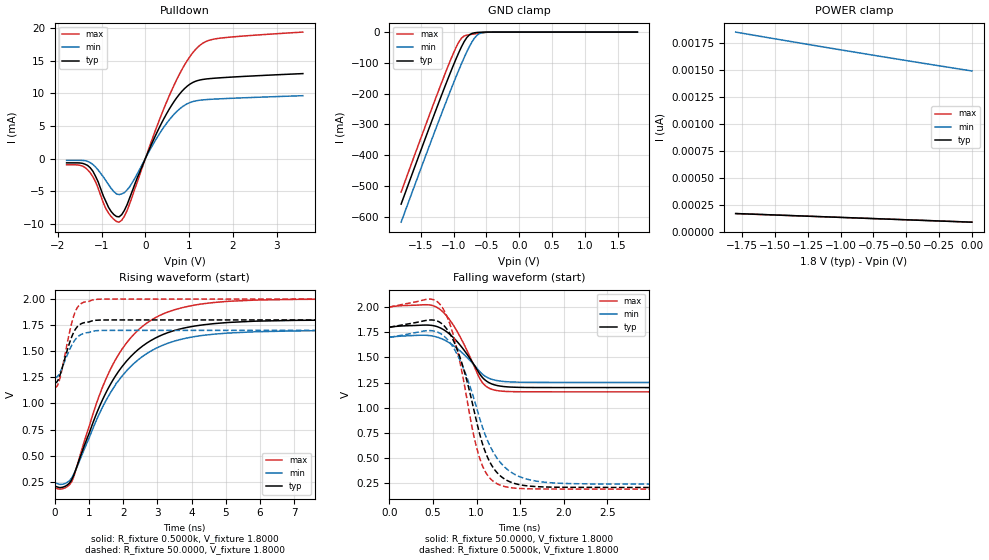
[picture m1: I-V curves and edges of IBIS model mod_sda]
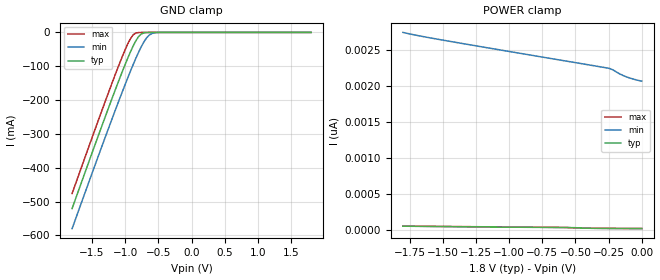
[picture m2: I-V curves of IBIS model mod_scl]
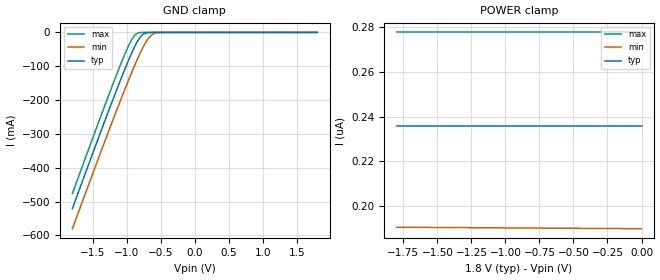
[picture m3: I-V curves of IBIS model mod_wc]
| IBIS (I/O, Buffer, Information, Specification) Model, officially
| electronic behavioral standard for Buffer structures of digital pins.
[IBIS ver]  4.0
[File name] m24c16_g1_tssop8.ibs
[File Rev]  0
[Date]   18 March 2015
[Source]   CAD & Design Services (Catania) - STMicroelectronics
[Notes]
   (Note1)  This IBIS model includes the TSSOP8 package data
   (Note2)  This IBIS model has some Notes about the non-monotonicity
   of the I-V curves, but they are not indicative of problems
   inside the model;
[Copyright] (c) 2015 STMicroelectronics
|   Component M24C16
[Component] M24C16
[Manufacturer] STMicroelectronics
[Package]
| variable  typ   min   max
R_pkg   0.0   0.0   0.0
L_pkg   0.0H   0.0H   0.0H
C_pkg   0.0F   0.0F   0.0F
[Pin]  signal_name   model_name   R_pin   L_pin   C_pin
1   NC   NC   NA   NA   NA
2   NC   NC   NA   NA   NA
3   NC   NC   NA   NA   NA
4   VSS   GND   NA   NA   NA
5   SDA   mod_sda   NA   NA   NA
6   SCL   mod_scl   NA   NA   NA
7   WCN   mod_wc   NA   NA   NA
8   VCC   POWER   NA   NA   NA
[Package Model]  182696_TSSOP8
[Define Package Model]  182696_TSSOP8
[Manufacturer]  STMicroelectronics
[OEM]  STMicroelectronics
[Description]  8 pin TSSOP package
[Number Of Pins]  8
[Pin Numbers]
|Pin Num   Terminal Name
1   | net1
2   | net2
3   | net3
4   | net4_GND
5   | net5
6   | net6
7   | net7
8   | net8_VDD
[Model Data]
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[End Model Data]
[End Package Model]
| Models and submodels in the file (3): mod_sda (I/O_open_drain), mod_scl (Input), mod_wc (Input)
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|   Model mod_sda
[Model]   mod_sda
Model_type I/O_open_drain
Polarity   Non-Inverting
Vinl   =   0.540V
Vinh   =   1.260V
Vmeas  =   0.900V
Cref   =   10pF
Rref   =   1k
Vref   =   1.800V
C_comp   2.668pF   2.547pF   2.925pF
[Temperature Range]  25.0000   0.1050k   -40.0000
[Voltage Range]   1.8000V   1.7000V   2.0000V
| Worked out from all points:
|   slope of the pulldown table from 0 to 0.27 V, typ, clamps not added: 66.3 ohm
|   GND clamp passes 1 mA (typ) near -0.63 V on its own axis
|   rising waveform, R_fixture 0.5000k, V_fixture 1.8000: 20-80 % time 1.53ns typ, 1.58ns min, 1.46ns max; typ from 0.207 V to 1.8 V
|   rising waveform, R_fixture 50.0000, V_fixture 1.8000: 20-80 % time 352ps typ, 384ps min, 337ps max; typ from 1.2 V to 1.8 V
|   falling waveform, R_fixture 50.0000, V_fixture 1.8000: 20-80 % time 297ps typ, 311ps min, 292ps max; typ from 1.8 V to 1.2 V
|   falling waveform, R_fixture 0.5000k, V_fixture 1.8000: 20-80 % time 300ps typ, 367ps min, 258ps max; typ from 1.8 V to 0.207 V
[Pulldown]
|Voltage   I(typ)   I(min)   I(max)
-1.8V     -665.8uA   -275.1uA   -956.4uA
-1.44V    -730.5uA   -283.4uA   -1.147mA
-1.26V    -1.416mA   -626uA     -2.177mA
-900mV    -6.632mA   -3.421mA   -7.74mA
-600mV    -8.957mA   -5.543mA   -9.785mA
-420mV    -7.139mA   -4.839mA   -8.038mA
60mV      953.5uA    767.3uA    1.16mA
480mV     6.822mA    5.362mA    8.599mA
840mV     10.37mA    7.928mA    13.73mA
1.14V     11.86mA    8.85mA     16.72mA
1.62V     12.37mA    9.153mA    18.42mA
3.6V      13.06mA    9.66mA     19.44mA
[GND_clamp]
|Voltage   I(typ)   I(min)   I(max)
-1.8V     -559.4mA   -618.2mA   -520.2mA
-1.2V     -214.3mA   -274.2mA   -173.7mA
-1.04V    -126.9mA   -186.2mA   -87.22mA
-960mV    -85.5mA    -143.6mA   -48.31mA
-880mV    -47.65mA   -102.7mA   -19.45mA
-800mV    -17.95mA   -64.52mA   -9.981mA
-760mV    -8.981mA   -47.2mA    -8.395mA
-720mV    -4.357mA   -31.76mA   -7.048mA
-640mV    -1.164mA   -9.757mA   -4.512mA
-560mV    -259.3uA   -1.789mA   -2.186mA
-440mV    -32.94uA   -178.5uA   -105.7uA
1.8V      87.14pA    1.509nA    78.96pA
[POWER_clamp]
|Voltage   I(typ)   I(min)   I(max)
-1.8V     167.6pA    1.851nA    166.7pA
-960mV    129.9pA    1.678nA    129.9pA
-480mV    108.5pA    1.583nA    108.8pA
0V        87.14pA    1.49nA     87.73pA
[Ramp]
| variable   typ   min   max
dV/dt_r   0.3599/0.4505n   0.2623/0.5115n   0.5053/0.3901n
dV/dt_f   0.3599/0.3419n   0.2623/0.3879n   0.5053/0.3191n
R_load = 50.0000
[Rising Waveform]   | New Temp 105 (min)
R_fixture= 0.5000k
V_fixture= 1.8000
V_fixture_min= 1.7000
V_fixture_max= 2.0000
|time   V(typ)   V(min)   V(max)
0s        207.5mV    240.5mV    191.1mV
310ps     206.8mV    234mV      192.3mV
510ps     279.3mV    293.7mV    260.1mV
1.27ns    941.6mV    877.8mV    1.047V
1.8ns     1.275V     1.193V     1.433V
2.33ns    1.485V     1.387V     1.668V
2.93ns    1.624V     1.523V     1.82V
3.77ns    1.721V     1.62V      1.921V
5.08ns    1.776V     1.674V     1.979V
10ns      1.8V       1.699V     2V
[Rising Waveform]
R_fixture= 50.0000
V_fixture= 1.8000   | New Temp (105)
V_fixture_min= 1.7000
V_fixture_max= 2.0000
|time   V(typ)   V(min)   V(max)
0s        1.2V       1.251V     1.158V
70ps      1.21V      1.255V     1.168V
150ps     1.269V     1.296V     1.24V
230ps     1.355V     1.355V     1.355V
450ps     1.597V     1.527V     1.709V
530ps     1.665V     1.577V     1.811V
610ps     1.714V     1.616V     1.887V
770ps     1.763V     1.66V      1.957V
1.11ns    1.792V     1.692V     1.992V
10ns      1.8V       1.7V       2V
[Falling Waveform]
R_fixture= 50.0000   | New Temp 105 (min)
V_fixture= 1.8000
V_fixture_min= 1.7000
V_fixture_max= 2.0000
|time   V(typ)   V(min)   V(max)
0s        1.8V       1.7V       2V
440ps     1.821V     1.718V     2.022V
580ps     1.794V     1.692V     1.977V
680ps     1.739V     1.649V     1.887V
780ps     1.654V     1.587V     1.754V
900ps     1.52V      1.491V     1.552V
1.06ns    1.308V     1.338V     1.258V
1.14ns    1.25V      1.294V     1.196V
1.28ns    1.214V     1.264V     1.165V
10ns      1.2V       1.251V     1.158V
[Falling Waveform]
R_fixture= 0.5000k   | New Temp 105 (Min)
V_fixture= 1.8000
V_fixture_min= 1.7000
V_fixture_max= 2.0000
|time   V(typ)   V(min)   V(max)
0s        1.8V       1.7V       2V
460ps     1.871V     1.766V     2.079V
610ps     1.829V     1.723V     1.993V
810ps     1.501V     1.473V     1.451V
970ps     978mV      1.09V      716.3mV
1.05ns    694.7mV    854.5mV    462.6mV
1.17ns    433.4mV    593.1mV    285.6mV
1.35ns    277.6mV    389.5mV    211.9mV
2.09ns    209.4mV    246.1mV    192.2mV
10ns      207.5mV    240.5mV    191.1mV
|   Model mod_scl
[Model]   mod_scl
Model_type Input
Vinl   =   0.540V
Vinh   =   1.260V
C_comp   2.119pF   2.024pF   2.323pF
[Temperature Range]  25.0000   0.1050k   -40.0000
[Voltage Range]   1.8000V   1.7000V   2.0000V
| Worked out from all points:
|   GND clamp passes 1 mA (typ) near -0.70 V on its own axis
[GND_clamp]
|Voltage   I(typ)   I(min)   I(max)
-1.8V     -520.9mA   -580.3mA   -476.5mA
-1.2V     -196.3mA   -256.7mA   -150.7mA
-1.04V    -114.2mA   -173.9mA   -69.64mA
-960mV    -75.5mA    -133.8mA   -33.44mA
-880mV    -40.19mA   -95.3mA    -7.264mA
-800mV    -12.93mA   -59.47mA   -439.4uA
-760mV    -5.118mA   -43.24mA   -158.9uA
-720mV    -1.576mA   -28.78mA   -102.3uA
-640mV    -136uA     -8.386mA   -70.17uA
-560mV    -28.62uA   -1.288mA   -47.23uA
-480mV    -12.31uA   -161.7uA   -26.66uA
1.8V      235.7nA    195.1nA    277.8nA
[POWER_clamp]
|Voltage   I(typ)   I(min)   I(max)
-1.8V     52.4pA     2.748nA    53.48pA
-1.68V    50.06pA    2.701nA    51.53pA
-1.5V     46.9pA     2.641nA    48.74pA
-580mV    32.98pA    2.352nA    35.02pA
-520mV    31.98pA    2.334nA    29.36pA
-260mV    20.67pA    2.253nA    22.45pA
-240mV    20.43pA    2.245nA    22.24pA
-220mV    20.21pA    2.229nA    22.04pA
-160mV    19.57pA    2.165nA    21.43pA
-120mV    19.17pA    2.133nA    21.03pA
-60mV     18.57pA    2.096nA    20.42pA
0V        17.97pA    2.069nA    19.82pA
|   Model mod_wc
[Model]   mod_wc
Model_type Input
Vinl   =   0.540V
Vinh   =   1.260V
C_comp   2.119pF   2.024pF   2.323pF
[Temperature Range]  25.0000   0.1050k   -40.0000
[Voltage Range]   1.8000V   1.7000V   2.0000V
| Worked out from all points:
|   GND clamp passes 1 mA (typ) near -0.70 V on its own axis
[GND_clamp]
|Voltage   I(typ)   I(min)   I(max)
-1.8V     -520.9mA   -580.3mA   -476.5mA
-1.2V     -196.3mA   -256.7mA   -150.7mA
-1.04V    -114.2mA   -173.9mA   -69.64mA
-960mV    -75.5mA    -133.8mA   -33.44mA
-880mV    -40.19mA   -95.3mA    -7.264mA
-800mV    -12.93mA   -59.47mA   -439.4uA
-760mV    -5.118mA   -43.24mA   -158.9uA
-720mV    -1.576mA   -28.78mA   -102.3uA
-640mV    -136uA     -8.386mA   -70.17uA
-560mV    -28.62uA   -1.288mA   -47.23uA
-480mV    -12.31uA   -161.7uA   -26.66uA
1.8V      3.236uA    3.19uA     3.278uA
[POWER_clamp]
|Voltage   I(typ)   I(min)   I(max)
-1.8V     235.7nA    190.4nA    277.8nA
-1.56V    235.7nA    190.4nA    277.8nA
-1.54V    235.7nA    190.3nA    277.8nA
-1.28V    235.7nA    190.3nA    277.8nA
-1.26V    235.7nA    190.2nA    277.8nA
-1.02V    235.7nA    190.2nA    277.8nA
-1V       235.7nA    190.1nA    277.8nA
-740mV    235.7nA    190.1nA    277.8nA
-720mV    235.7nA    190nA      277.8nA
-460mV    235.7nA    190nA      277.8nA
-440mV    235.7nA    189.9nA    277.8nA
0V        235.7nA    189.8nA    277.8nA
